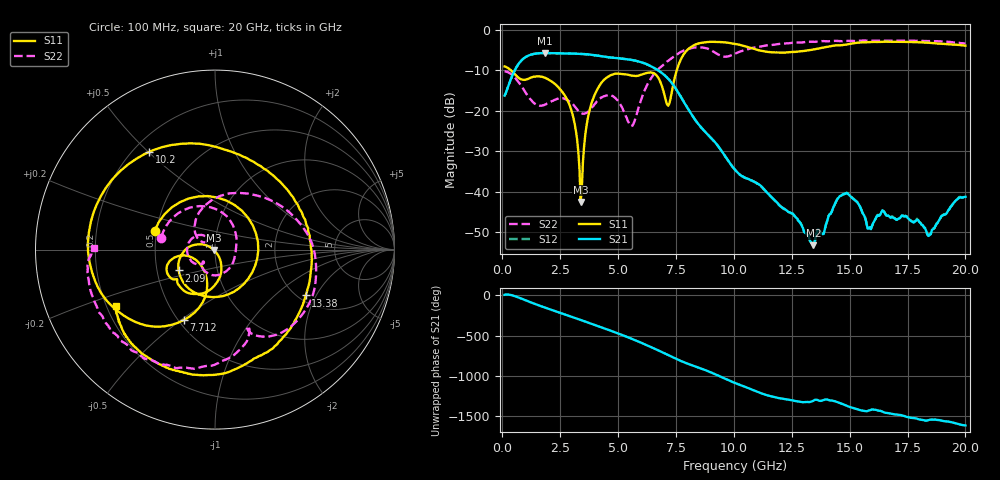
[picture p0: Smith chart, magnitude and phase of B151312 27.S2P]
!  2-Port S-parameters saved by WinCal
! VAR MeasName=S-Parameters (CALIBRATED_DATA) read from VNA (N5244A)
! VAR MeasDate=12/8/2015 5:45:29 PM
! VAR NAME=B151312 27
! VAR FILENAME=B151312 27.S2P
! VAR DATE=12/8/2015 5:45:29 PM
! VAR PHYS_PORTS=1,2
# Hz S DB R 50
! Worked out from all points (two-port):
!   401 points, 100 MHz to 20 GHz, reference 50 ohm
!   highest |S21| = -5.76 dB at 1.841 GHz (marker M1); lowest = -53.2 dB at 13.43 GHz (marker M2)
!   |S21| within 3 dB of the highest: 665 MHz to 6.332 GHz (5.667 GHz wide, 162 % of centre)
!   lowest |S11| = -42.5 dB at 3.384 GHz (marker M3), VSWR 1.02, Z = 49.3 - j0.146 ohm
!   |S11| at or under -10 dB: 368.6 MHz to 7.536 GHz (7.167 GHz wide, 181 % of centre)
!   |S22| runs from -23.8 to -2.6 dB; largest |S21 - S12| = 0.0014
!   S11 on the Smith chart (normalised r, x): 100 MHz: 0.49, +0.12; 2.09 GHz: 0.65, -0.16; 7.712 GHz: 0.53, -0.51; 10.2 GHz: 0.26, +0.50; 13.38 GHz: 2.19, -1.65; 20 GHz: 0.24, -0.25
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1e8  -9.06 162.6  -16.27 7.2  -16.26 7.2  -10.25 167.4
8.4625e8  -12.29 10.1  -7.48 -42.6  -7.48 -42.6  -14.05 71.5
1.84125e9  -11.85 -132.2  -5.76 -151.5  -5.76 -151.5  -18.48 -25.3
2.09e9  -12.64 -150.2  -5.78 -176.5  -5.78 -176.5  -17.80 -47.7
2.93575e9  -19.06 165.7  -5.88 100.3  -5.88 100.3  -17.82 -120.9
3.3835e9  -42.51 -168.6  -5.96 55.3  -5.96 55.3  -20.51 -135.0
3.43325e9  -39.26 -81.6  -5.98 50.3  -5.98 50.2  -20.64 -135.2
3.73175e9  -20.81 -67.9  -6.10 19.6  -6.11 19.6  -20.17 -130.3
4.32875e9  -12.77 -98.3  -6.58 -41.9  -6.58 -41.9  -16.60 -156.8
5.5725e9  -11.31 -140.7  -7.43 -176.6  -7.44 -176.7  -23.78 135.4
6.7665e9  -12.15 -167.4  -10.16 33.5  -10.17 33.4  -9.58 71.7
7.1645e9  -18.75 -137.4  -12.11 -21.0  -12.08 -21.1  -7.67 41.8
7.71175e9  -7.34 -113.9  -16.59 -93.9  -16.54 -94.0  -5.48 6.5
8.80625e9  -3.07 -174.6  -25.47 148.3  -25.45 148.0  -4.56 -52.0
1.005e10  -3.49 130.8  -34.54 -7.0  -34.61 -7.0  -5.93 -68.0
1.019925e10  -3.66 123.9  -35.45 -23.6  -35.51 -23.9  -5.55 -69.6
1.338325e10  -4.94 -26.8  -52.74 126.0  -52.70 125.2  -2.99 -117.6
1.3433e10  -4.89 -28.4  -53.22 132.1  -53.42 133.4  -3.01 -118.5
1.477625e10  -3.72 -72.2  -40.54 82.5  -40.59 82.9  -2.81 -134.3
1.67165e10  -2.99 -113.5  -46.09 -24.8  -45.86 -25.0  -2.68 -151.8
1.845775e10  -3.24 -137.0  -50.59 -103.2  -50.68 -103.5  -2.81 -167.2
2e10  -3.94 -150.3  -41.23 -174.0  -41.19 -175.2  -3.42 179.3
